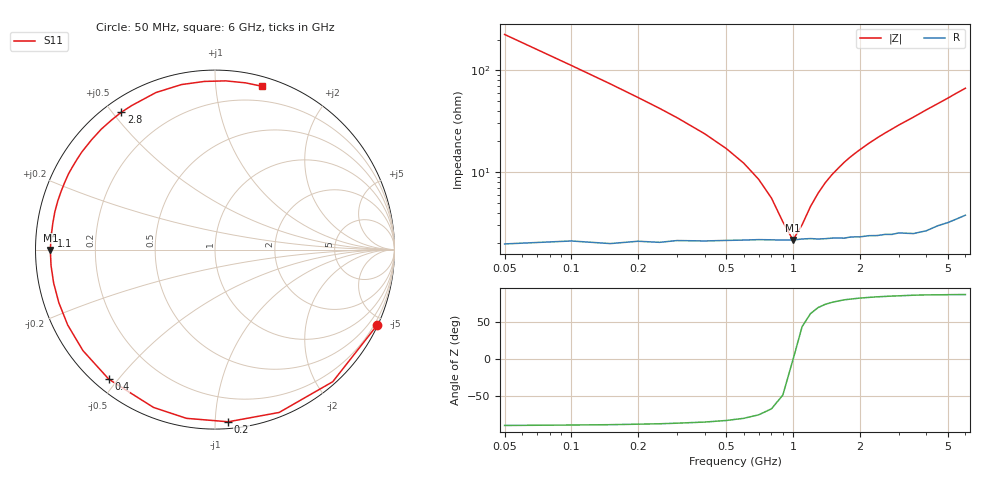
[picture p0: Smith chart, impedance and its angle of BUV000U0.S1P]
! Infineon Technologies  Discrete & RF Semiconductors
! BB 833
! Si Tuning Diode in SOD323
! VR = 0 V
! S-Parameters:  June  1999
# GHz  S  MA  R  50
!  f  S11
! GHz  MAG  ANG
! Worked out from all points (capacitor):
!   34 points, 50 MHz to 6 GHz, reference 50 ohm
!   read as one part to ground: C = 14.1 pF near 50 MHz
!   lowest |Z| = 2.15 ohm at 1 GHz (marker M1)
!   series resonance near 1.002 GHz, so ESL is about 1.8 nH
!   S11 on the Smith chart (normalised r, x): 50 MHz: 0.04, -4.49; 200 MHz: 0.04, -1.08; 400 MHz: 0.04, -0.47; 1.1 GHz: 0.04, +0.04; 2.8 GHz: 0.05, +0.53; 6 GHz: 0.08, +1.33
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0.05  0.9963 -25.1
0.1  0.986 -48.3
0.15  0.9752 -68.5
0.2  0.9621 -85.6
0.25  0.9535 -99.6
0.3  0.9437 -111.3
0.4  0.9335 -129.3
0.5  0.9263 -142.6
0.6  0.922 -152.9
0.7  0.919 -161.3
0.8  0.918 -168.3
0.9  0.9178 -174.4
1  0.9175 -179.9
1.1  0.9159 175.2
1.2  0.9154 170.8
1.4  0.9169 162.8
1.6  0.9173 155.9
1.8  0.9182 149.4
2  0.92 143.7
2.4  0.9229 133.3
2.8  0.9264 124.3
3  0.927 120.0
3.5  0.9349 110.6
4  0.9383 101.5
4.5  0.9388 93.6
5  0.9419 86.4
5.5  0.9446 79.6
6  0.947 73.8
